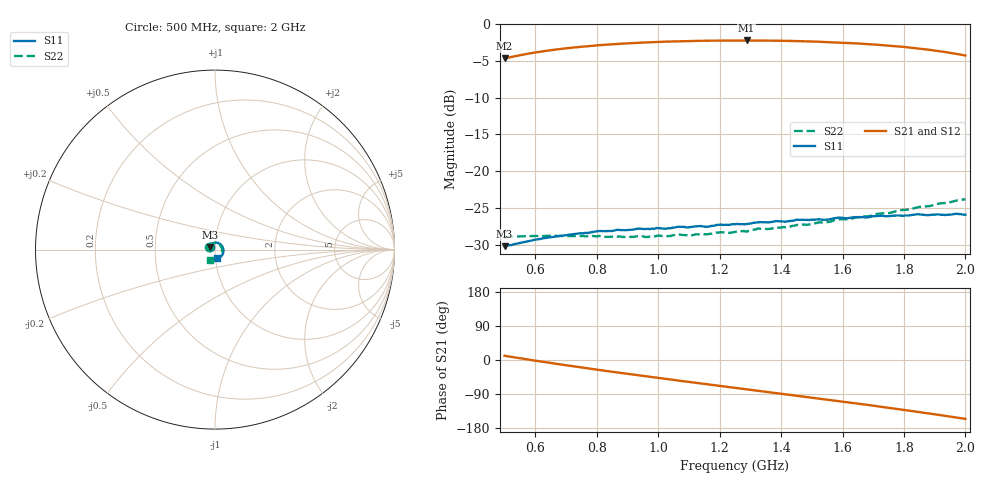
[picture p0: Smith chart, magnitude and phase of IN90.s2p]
!Agilent Technologies,E8363B,SG43030131,A.07.50.48
!Agilent E8363B: A.07.50.48
!Date: Thursday, October 16, 2025 22:14:58
!Correction: S11(Full 2 Port(1,2))
!S21(Full 2 Port(1,2))
!S12(Full 2 Port(1,2))
!S22(Full 2 Port(1,2))
!S2P File: Measurements: S11, S21, S12, S22:
# Hz S  dB  R 50
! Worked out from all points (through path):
!   201 points, 500 MHz to 2 GHz, reference 50 ohm
!   highest |S21| = -2.21 dB at 1.288 GHz (marker M1); lowest = -4.7 dB at 500 MHz (marker M2)
!   lowest |S11| = -30.2 dB at 500 MHz (marker M3), VSWR 1.06, Z = 47.3 + j1.36 ohm
!   |S11| at or under -10 dB: start of sweep to end of sweep
!   |S22| runs from -29.0 to -23.8 dB; largest |S21 - S12| = 0.0016
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5e8  -30.20 152.4  -4.66 11.1  -4.67 11.1  -28.98 158.5
5.675e8  -29.61 136.0  -4.08 2.3  -4.09 2.3  -28.84 143.7
6.2e8  -29.18 124.5  -3.72 -4.2  -3.73 -4.3  -28.83 132.3
6.875e8  -28.77 111.5  -3.34 -12.4  -3.35 -12.4  -28.82 118.1
7.55e8  -28.46 99.2  -3.05 -20.3  -3.06 -20.3  -28.80 103.8
8.675e8  -27.96 82.3  -2.69 -33.0  -2.69 -33.0  -28.89 81.1
9.65e8  -27.84 67.5  -2.47 -43.6  -2.48 -43.6  -28.95 61.9
1.0025e9  -27.76 62.4  -2.41 -47.6  -2.42 -47.5  -28.76 54.7
1.07e9  -27.57 52.8  -2.32 -54.7  -2.33 -54.7  -28.63 42.3
1.1e9  -27.64 49.4  -2.29 -57.9  -2.30 -57.8  -28.79 36.6
1.13e9  -27.48 45.4  -2.27 -60.9  -2.28 -61.0  -28.59 30.5
1.25e9  -27.22 30.7  -2.21 -73.3  -2.22 -73.4  -28.26 10.1
1.2875e9  -27.21 25.4  -2.21 -77.2  -2.23 -77.2  -28.22 2.3
1.325e9  -26.94 21.1  -2.22 -81.0  -2.23 -81.0  -27.80 -3.2
1.4e9  -26.83 12.3  -2.26 -88.8  -2.27 -88.8  -27.67 -16.3
1.505e9  -26.59 1.2  -2.36 -99.6  -2.37 -99.6  -27.15 -32.5
1.6325e9  -26.29 -14.7  -2.59 -113.1  -2.59 -113.1  -26.42 -52.8
1.7525e9  -26.12 -31.3  -2.92 -126.3  -2.93 -126.3  -25.69 -72.7
1.8425e9  -25.86 -46.0  -3.28 -136.5  -3.29 -136.5  -24.93 -86.9
1.88e9  -25.98 -51.8  -3.47 -140.9  -3.47 -140.9  -24.76 -93.5
1.9475e9  -25.91 -64.5  -3.88 -149.0  -3.88 -149.0  -24.26 -105.1
2e9  -25.92 -75.9  -4.26 -155.4  -4.27 -155.4  -23.80 -114.7
